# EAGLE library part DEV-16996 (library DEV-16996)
Development Boards & Kits - ARM ,, Source: Datasheet
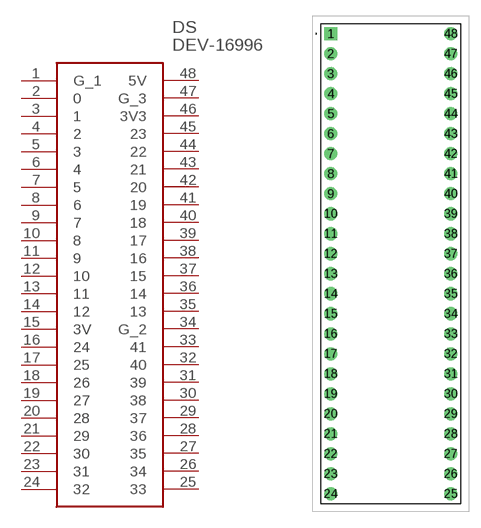
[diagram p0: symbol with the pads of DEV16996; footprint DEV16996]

Designator prefix DS

## DEV-16996 (Arrow_Part_Number: DEV-16996; Arrow_Price-Stock: https://www.arrow.com/en/products/dev-16996/sparkfun-electronics?region=nac; Description: Development Boards & Kits - ARM ,,; Height: 4.1mm; Manufacturer_Name: SparkFun; Manufacturer_Part_Number: DEV-16996; Mouser_Part_Number: 474-DEV-16996; Mouser_Price-Stock: https://www.mouser.co.uk/ProductDetail/SparkFun/DEV-16996?qs=hWgE7mdIu5Su1vq701B2Wg%3D%3D)  [DEV16996]
1  G_1
2  0
3  1
4  2
5  3
6  4
7  5
8  6
9  7
10  8
11  9
12  10
13  11
14  12
15  3V
16  24
17  25
18  26
19  27
20  28
21  29
22  30
23  31
24  32
25  33
26  34
27  35
28  36
29  37
30  38
31  39
32  40
33  41
34  G_2
35  13
36  14
37  15
38  16
39  17
40  18
41  19
42  20
43  21
44  22
45  23
46  3V3
47  G_3
48  5V

## Footprint DEV16996 (pad centres in mm)
DEV-16996-1
drill 1.11 pad 1.665 square: 1 0,0
drill 1.11 pad 1.665: 2 0,-2.54; 3 0,-5.08; 4 0,-7.62; 5 0,-10.16; 6 0,-12.7; 7 0,-15.24; 8 0,-17.78; 9 0,-20.32; 10 0,-22.86; 11 0,-25.4; 12 0,-27.94; 13 0,-30.48; 14 0,-33.02; 15 0,-35.56; 16 0,-38.1; 17 0,-40.64; 18 0,-43.18; 19 0,-45.72; 20 0,-48.26; 21 0,-50.8; 22 0,-53.34; 23 0,-55.88; 24 0,-58.42; 25 15.24,-58.42; 26 15.24,-55.88; 27 15.24,-53.34; 28 15.24,-50.8; 29 15.24,-48.26; 30 15.24,-45.72; 31 15.24,-43.18; 32 15.24,-40.64; 33 15.24,-38.1; 34 15.24,-35.56; 35 15.24,-33.02; 36 15.24,-30.48; 37 15.24,-27.94; 38 15.24,-25.4; 39 15.24,-22.86; 40 15.24,-20.32; 41 15.24,-17.78; 42 15.24,-15.24; 43 15.24,-12.7; 44 15.24,-10.16; 45 15.24,-7.62; 46 15.24,-5.08; 47 15.24,-2.54; 48 15.24,0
